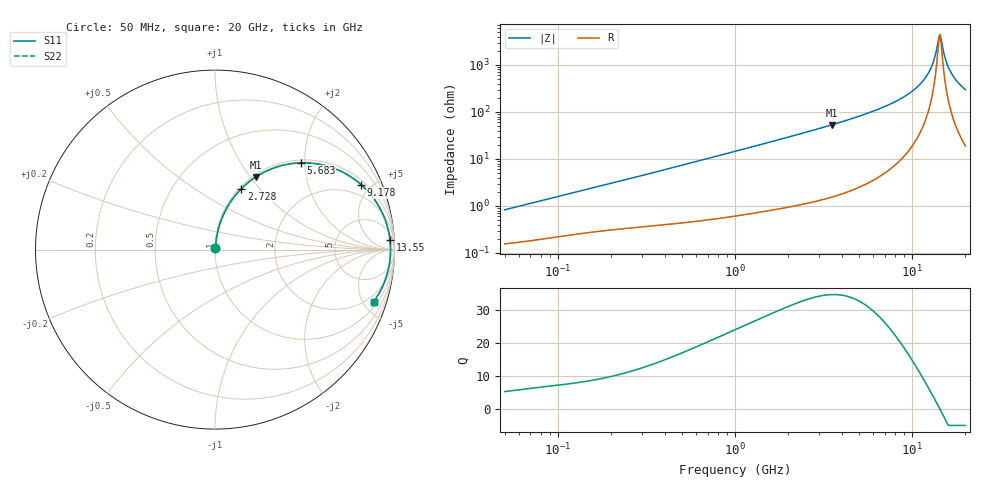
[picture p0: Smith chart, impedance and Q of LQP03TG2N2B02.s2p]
!Murata Part Number: LQP03TG2N2B02
!These Parameters are Measured in Series Mode Connection
!  o--[Z]--o
!Port1  Port2
!  o-------o
!Freq. Start=50[MHz] Stop=20[GHz], 401[Steps]
# Hz S RI R 50
!Freq.(Hz) S11(Real) S11(Imag) S21(Real) S21(Imag) S12(Real) S12(Imag) S22(Real) S22(Imag)
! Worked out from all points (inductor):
!   401 points, 50 MHz to 20 GHz, reference 50 ohm
!   read as one part in series: L = 2.56 nH near 51.52 MHz
!   highest Q = 34.5 at 3.519 GHz (marker M1), where L = 2.4 nH
!   self-resonance near 14.17 GHz
!   S11 on the Smith chart (normalised r, x): 50 MHz: 1.00, +0.02; 2.728 GHz: 1.02, +0.81; 5.683 GHz: 1.06, +1.91; 9.178 GHz: 1.25, +4.39; 13.55 GHz: 13, +31; 20 GHz: 1.38, -5.97
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5e7  0.00162 0.00811  0.9984 -0.00811  0.9984 -0.00811  0.00162 0.00811
1.364002e8  0.00303 0.0209  0.997 -0.0209  0.997 -0.0209  0.00303 0.0209
3.721004e8  0.00682 0.0543  0.9932 -0.0543  0.9932 -0.0543  0.00682 0.0543
1e9  0.0263 0.1403  0.9737 -0.1403  0.9737 -0.1403  0.0263 0.1403
1.766834e9  0.0688 0.2369  0.9312 -0.2369  0.9312 -0.2369  0.0688 0.2369
2.728004e9  0.1469 0.3394  0.8531 -0.3394  0.8531 -0.3394  0.1469 0.3394
3.519108e9  0.227 0.4047  0.773 -0.4047  0.773 -0.4047  0.227 0.4047
5.683258e9  0.4776 0.4835  0.5224 -0.4835  0.5224 -0.4835  0.4776 0.4835
7.442007e9  0.6684 0.4508  0.3316 -0.4508  0.3316 -0.4508  0.6684 0.4508
9.178299e9  0.8149 0.3612  0.1851 -0.3612  0.1851 -0.3612  0.8149 0.3612
1.066139e10  0.9008 0.2609  0.0992 -0.2609  0.0992 -0.2609  0.9008 0.2609
1.183995e10  0.9445 0.1756  0.0555 -0.1756  0.0555 -0.1756  0.9445 0.1756
1.276073e10  0.9653 0.109  0.0347 -0.109  0.0347 -0.109  0.9653 0.109
1.354865e10  0.975 0.0536  0.025 -0.0536  0.025 -0.0536  0.975 0.0536
1.396067e10  0.9774 0.0255  0.0226 -0.0255  0.0226 -0.0255  0.9774 0.0255
1.417136e10  0.978 0.0114  0.022 -0.0114  0.022 -0.0114  0.978 0.0114
1.438523e10  0.9782 -0.00272  0.0218 0.00272  0.0218 0.00272  0.9782 -0.00272
1.460232e10  0.978 -0.0168  0.022 0.0168  0.022 0.0168  0.978 -0.0168
1.573793e10  0.9708 -0.087  0.0292 0.087  0.0292 0.087  0.9708 -0.087
1.646126e10  0.9616 -0.1281  0.0384 0.1281  0.0384 0.1281  0.9616 -0.1281
1.800918e10  0.9332 -0.2067  0.0668 0.2067  0.0668 0.2067  0.9332 -0.2067
2e10  0.8847 -0.2892  0.1153 0.2892  0.1153 0.2892  0.8847 -0.2892
